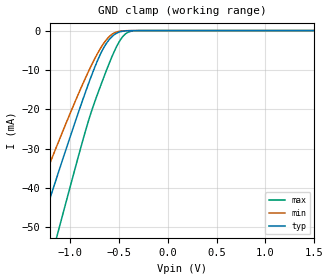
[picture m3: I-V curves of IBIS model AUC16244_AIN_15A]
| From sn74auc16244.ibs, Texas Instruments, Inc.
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[Model]   AUC16244_AIN_15A
Model_type  Input
Vinl=0.49
Vinh=1.04
| variable   typ   min   max
C_comp   3.30pF   2.62pF   3.86pF
[Temperature Range]   40   100   -40
| Ambient temperature   25   85   -40
[Voltage range]   1.5   1.4   1.6
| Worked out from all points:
|   GND clamp passes 1 mA (typ) near -0.54 V on its own axis
[GND Clamp]
| AUC16244_AIN_15A
|   Voltage   I(typ)   I(min)   I(max)
-3.6V     -231.9mA   -193.8mA   -279.4mA
-1.47V    -63.37mA   -50.63mA   -83.77mA
-1.335V   -52.84mA   -41.98mA   -71.19mA
-1.295V   -49.73mA   -39.44mA   -67.46mA
-1.13V    -37.04mA   -29.11mA   -52.07mA
-1.08V    -33.24mA   -26.05mA   -47.41mA
-815mV    -13.9mA    -10.68mA   -23.37mA
-695mV    -6.389mA   -4.864mA   -14.65mA
-575mV    -1.685mA   -1.059mA   -6.96mA
-430mV    -77.57uA   -37uA      -820.2uA
-280mV    -828.9nA   -591.8nA   -5.688uA
1.5V      179pA      278.7pA    184.7pA
